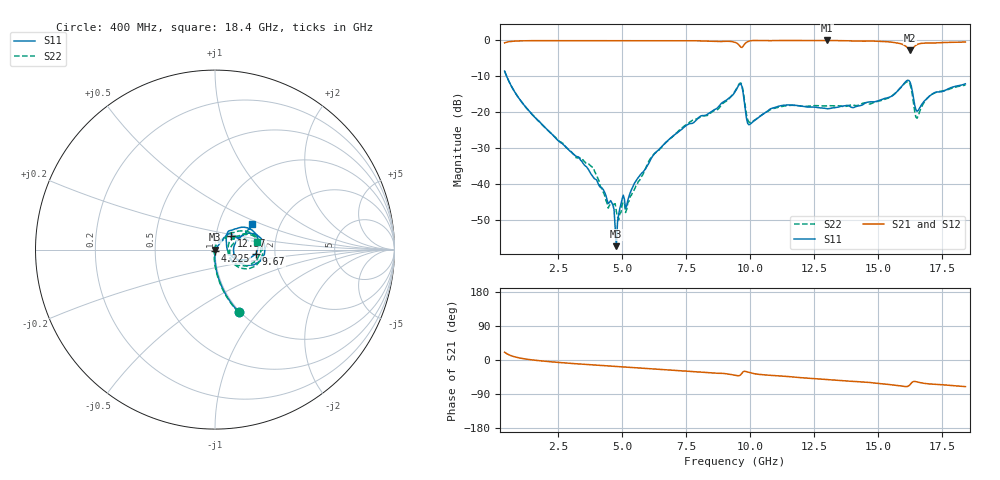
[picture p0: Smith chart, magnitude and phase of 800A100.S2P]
!  American Technical Ceramics  Date:  9/12/2007
!  One Norden Lane
!  Huntington Station,  NY.  11746-2102
!  Tel:  (631) 622-4700  Fax:  (631) 622-4748
!  Part Number  800A100  Mounting Orientation: Vertical
!  Description: Ultra Low ESR Microwave capacitors
!  Application: Coupling, Bypass, Tuning, DC Block
!  Filters, Matching
# GHZ S DB R 50
! Freq  |S11|  S11 Ph  |S21|  S21 Ph  |S12|  S12 Ph  |S22|  S22 Ph
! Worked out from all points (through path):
!   401 points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, 400 MHz to 18.4 GHz, reference 50 ohm
!   highest |S21| = 0.00 dB at 13 GHz (marker M1); lowest = -2.7 dB at 16.24 GHz (marker M2)
!   group delay of S21, straight-line fit = 11.8 ps
!   lowest |S11| = -57.3 dB at 4.765 GHz (marker M3), VSWR 1.00, Z = 50.1 - j0.018 ohm
!   |S11| at or under -10 dB: 481.2 MHz to end of sweep
!   |S22| runs from -50.0 to -8.6 dB; largest |S21 - S12| = 0.0022
!   S11 on the Smith chart (normalised r, x): 400 MHz: 0.99, -0.80; 4.225 GHz: 1.00, -0.02; 9.67 GHz: 1.59, -0.08; 12.37 GHz: 1.19, +0.18; 18.4 GHz: 1.44, +0.43
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0.4  -8.55 -69.0  -0.67 20.6  -0.67 20.6  -8.56 -69.4
1.39  -19.93 -87.2  -0.07 1.0  -0.07 1.0  -19.95 -88.7
3.415  -33.68 -100.5  -0.05 -10.9  -0.06 -10.9  -33.33 -93.3
3.865  -38.10 -100.0  -0.06 -13.1  -0.06 -13.0  -35.31 -109.5
4.225  -41.31 -92.7  -0.05 -14.7  -0.06 -14.7  -42.01 -120.2
4.585  -45.17 -74.4  -0.04 -16.4  -0.05 -16.3  -45.77 -130.5
4.765  -57.32 -7.6  -0.06 -17.1  -0.06 -17.1  -47.67 155.1
4.99  -44.20 6.1  -0.06 -18.2  -0.06 -18.2  -45.71 103.5
5.215  -44.48 26.1  -0.05 -19.1  -0.06 -19.1  -45.19 88.0
6.43  -30.39 51.1  -0.05 -24.4  -0.05 -24.4  -30.54 70.4
9.4  -14.33 40.4  -0.53 -40.3  -0.52 -40.2  -14.13 31.6
9.67  -12.77 -5.9  -1.96 -34.8  -1.96 -34.8  -12.44 -15.4
9.985  -23.37 17.0  -0.12 -33.5  -0.12 -33.5  -22.88 -1.6
11.11  -18.32 48.1  -0.02 -41.8  -0.01 -41.8  -18.58 31.4
12.37  -18.55 39.1  -0.01 -48.6  -0.01 -48.6  -18.23 32.2
12.415  -18.57 38.9  -0.01 -48.8  -0.01 -48.8  -18.23 32.3
13  -19.02 37.0  0.00 -51.7  -0.01 -51.7  -18.22 33.2
15.43  -15.81 26.6  -0.42 -64.8  -0.41 -64.8  -15.90 29.7
16.24  -11.65 -13.7  -2.71 -64.9  -2.69 -64.9  -12.26 -22.2
16.51  -19.74 -1.9  -1.14 -57.7  -1.14 -57.7  -21.65 -2.9
17.095  -14.98 27.4  -0.71 -63.6  -0.71 -63.6  -15.03 18.9
18.4  -12.09 34.5  -0.44 -70.2  -0.42 -70.2  -12.45 10.2
